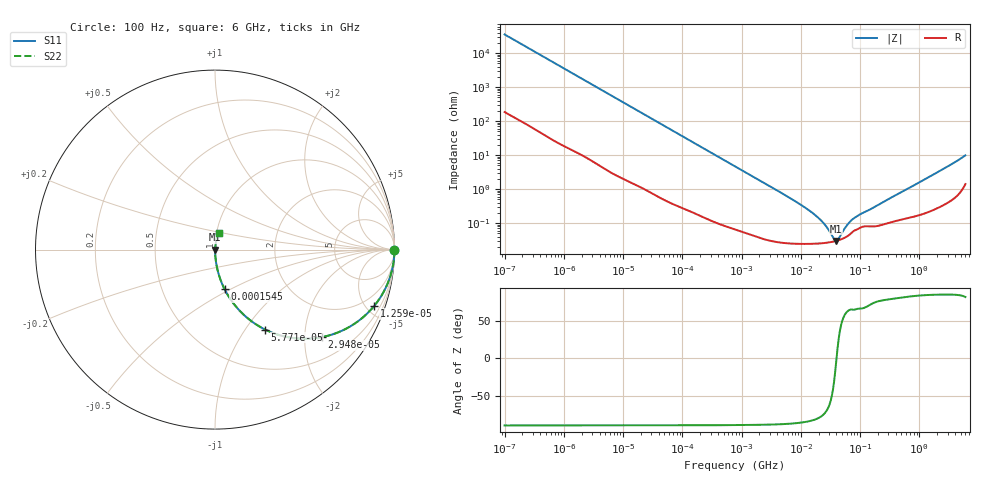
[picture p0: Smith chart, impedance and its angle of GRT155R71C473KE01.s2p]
!Murata Part Number: GRT155R71C473KE01
!These Parameters are Measured in Series Mode Connection
!Data Generated on Jun 19, 2026
!  o--ll--o
!Port1  Port2
!  o------o
!Operation Temp=25[degC], DC Bias Voltage=0[V]
!Freq. Start=100[Hz] Stop=6[GHz] 401[Steps]
# Hz S RI R 50
!Freq.(Hz) S11(Real) S11(Imag) S21(Real) S21(Imag) S12(Real) S12(Imag) S22(Real) S22(Imag)
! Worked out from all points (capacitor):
!   401 points, 100 Hz to 6 GHz, reference 50 ohm
!   read as one part in series: C = 45.4 nF near 109 Hz
!   lowest |Z| = 30 mohm at 39.84 MHz (marker M1)
!   series resonance near 40.09 MHz, so ESL is about 350 pH
!   S11 on the Smith chart (normalised r, x): 100 Hz: open; 12.59 kHz: 1.03, -5.66; 29.48 kHz: 1.02, -2.42; 57.71 kHz: 1.01, -1.24; 154.5 kHz: 1.00, -0.47; 6 GHz: 1.03, +0.19
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100  1 -0.00285  2.31e-05 0.00285  2.31e-05 0.00285  1 -0.00285
2008  0.9965 -0.0565  0.00353 0.0565  0.00353 0.0565  0.9965 -0.0565
5378  0.9768 -0.1478  0.0232 0.1478  0.0232 0.1478  0.9768 -0.1478
12592  0.8874 -0.3132  0.1126 0.3132  0.1126 0.3132  0.8874 -0.3132
18841  0.7804 -0.4109  0.2196 0.4109  0.2196 0.4109  0.7804 -0.4109
29482  0.5944 -0.4878  0.4056 0.4878  0.4056 0.4878  0.5944 -0.4878
40335  0.4407 -0.4932  0.5593 0.4932  0.5593 0.4932  0.4407 -0.4932
57709  0.2795 -0.4454  0.7205 0.4454  0.7205 0.4454  0.2795 -0.4454
90302  0.1382 -0.3414  0.8618 0.3414  0.8618 0.3414  0.1382 -0.3414
154540  0.0531 -0.22  0.9469 0.22  0.9469 0.22  0.0531 -0.22
316350  0.014 -0.1124  0.986 0.1124  0.986 0.1124  0.014 -0.1124
774597  0.00283 -0.0467  0.9972 0.0467  0.9972 0.0467  0.00283 -0.0467
6353432  0.000283 -0.00562  0.9997 0.00562  0.9997 0.00562  0.000283 -0.00562
1.555665e7  0.000249 -0.002  0.9998 0.002  0.9998 0.002  0.000249 -0.002
2.327686e7  0.000257 -0.00104  0.9997 0.00104  0.9997 0.00104  0.000257 -0.00104
3.64232e7  0.000288 -0.000175  0.9997 0.000175  0.9997 0.000175  0.000288 -0.000175
3.983537e7  0.000299 -1.14e-05  0.9997 1.14e-05  0.9997 1.14e-05  0.000299 -1.14e-05
4.35672e7  0.000313 0.000152  0.9997 -0.000152  0.9997 -0.000152  0.000313 0.000152
6.233367e7  0.00042 0.000829  0.9996 -0.000829  0.9996 -0.000829  0.00042 0.000829
7.797396e7  0.000584 0.00124  0.9994 -0.00124  0.9994 -0.00124  0.000584 0.00124
3.124326e8  0.00105 0.00514  0.999 -0.00514  0.999 -0.00514  0.00105 0.00514
6e9  0.0228 0.0935  0.9772 -0.0935  0.9772 -0.0935  0.0228 0.0935
